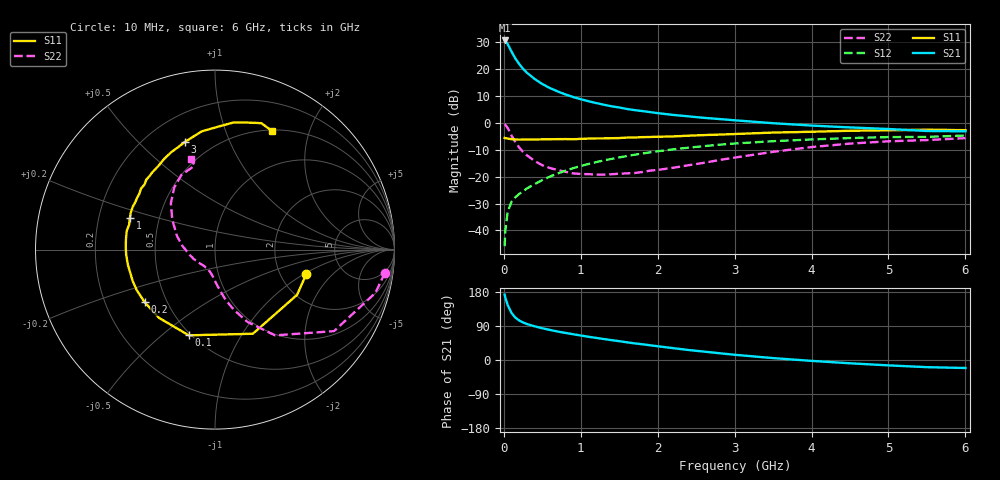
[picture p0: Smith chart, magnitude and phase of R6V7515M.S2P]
! SIEMENS Small Signal Semiconductors
! BFR193
! Si NPN RF Bipolar Junction Transistor in SOT23
! VCE = 0.75 V  IC = 15 mA
! Common Emitter S-Parameters:  May  1996
# GHz  S  MA  R  50
!  f  S11  S21  S12  S22
! GHz  MAG  ANG  MAG  ANG  MAG  ANG  MAG  ANG
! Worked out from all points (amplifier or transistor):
!   36 points, 10 MHz to 6 GHz, reference 50 ohm
!   highest |S21| = 30.7 dB at 10 MHz (marker M1)
!   |S21| within 3 dB of that: start of sweep to 79.17 MHz
!   unconditionally stable (mu >= 1): 563.5 MHz to 2.289 GHz
!   at 250 MHz: K = 0.78, MSG = 22.8 dB, |S12| = -25.4 dB
!   at 1.4 GHz: K = 1.05, MAG = 8.5 dB, |S12| = -13.4 dB
!   at 6 GHz: K = 0.98, MSG = 0.8 dB, |S12| = -4.7 dB
!   S11 on the Smith chart (normalised r, x): 10 MHz: 2.78, -1.05; 100 MHz: 0.49, -0.62; 200 MHz: 0.38, -0.29; 1 GHz: 0.34, +0.16; 3 GHz: 0.35, +0.70; 6 GHz: 0.51, +1.46
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0.01  0.5267 -15.0  34.31 172.3  0.0051 84.1  0.9558 -7.7
0.02  0.5221 -28.9  33.51 164.4  0.0101 78.8  0.9257 -15.1
0.05  0.5141 -65.8  29.3 145.0  0.0223 67.3  0.8039 -34.4
0.1  0.4994 -107.0  21.25 124.1  0.0342 57.0  0.5834 -55.0
0.15  0.4919 -129.3  15.84 111.8  0.0416 54.3  0.4407 -65.9
0.2  0.4895 -143.2  12.5 104.3  0.0478 55.4  0.3488 -72.8
0.25  0.4912 -152.7  10.17 98.9  0.0538 57.1  0.2888 -77.8
0.3  0.4907 -159.4  8.599 95.0  0.0604 58.1  0.2499 -81.0
0.4  0.4928 -170.2  6.591 88.9  0.073 60.9  0.1966 -86.9
0.5  0.496 -176.9  5.301 83.7  0.0865 62.1  0.1633 -92.1
0.6  0.4975 177.6  4.455 79.3  0.1008 62.9  0.1448 -96.0
0.7  0.5 172.5  3.862 75.1  0.1149 63.2  0.1331 -100.0
0.8  0.5025 168.1  3.397 71.5  0.1293 62.9  0.1234 -104.6
1  0.5059 159.7  2.767 64.6  0.1582 62.0  0.1124 -113.6
1.1  0.5124 156.4  2.539 61.3  0.1727 61.1  0.1117 -118.4
1.6  0.5344 140.5  1.822 46.6  0.2422 55.2  0.1156 -141.9
2.2  0.5622 124.4  1.412 31.3  0.3227 46.6  0.1466 -169.2
3  0.6227 105.7  1.122 13.8  0.4148 33.9  0.2268 159.8
3.5  0.6628 96.4  0.99 5.0  0.458 25.9  0.2904 145.0
4.5  0.7163 81.6  0.826 -8.7  0.5244 11.7  0.4131 123.4
5.5  0.7502 69.9  0.709 -18.9  0.552 -1.9  0.4807 103.8
6  0.7343 64.6  0.7 -21.1  0.584 -5.9  0.5216 104.6
